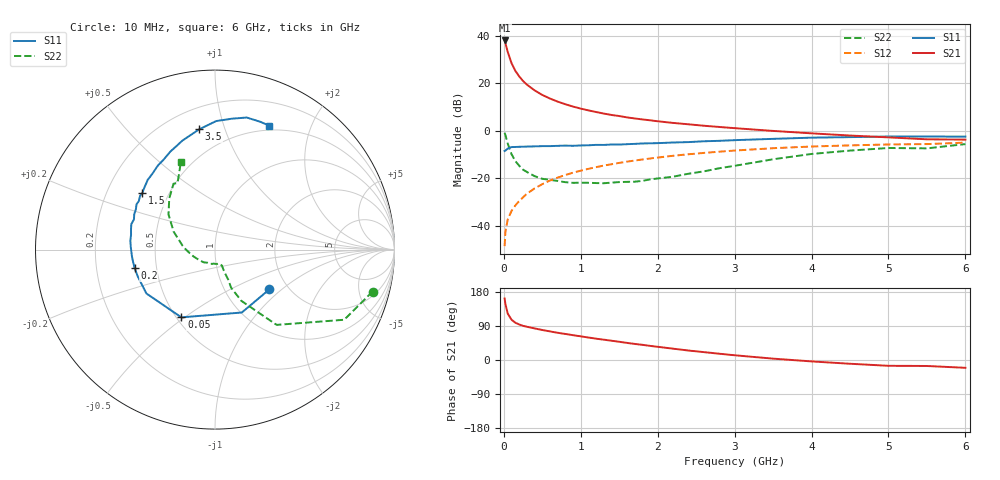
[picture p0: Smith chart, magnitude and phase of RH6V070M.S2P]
! SIEMENS Small Signal Semiconductors
! BFR106
! Si NPN RF Bipolar Junction Transistor in SOT23
! VCE = 6 V  IC = 70 mA
! Common Emitter S-Parameters:  August  1996
# GHz  S  MA  R  50
!  f  S11  S21  S12  S22
! GHz  MAG  ANG  MAG  ANG  MAG  ANG  MAG  ANG
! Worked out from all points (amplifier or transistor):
!   36 points, 10 MHz to 6 GHz, reference 50 ohm
!   highest |S21| = 38.1 dB at 10 MHz (marker M1)
!   |S21| within 3 dB of that: start of sweep to 35.63 MHz
!   unconditionally stable (mu >= 1): 213.4 MHz to 2.336 GHz
!   at 250 MHz: K = 1.03, MAG = 23.4 dB, |S12| = -28.0 dB
!   at 1.4 GHz: K = 1.06, MAG = 8.9 dB, |S12| = -14.1 dB
!   at 6 GHz: K = 0.99, MSG = 0.6 dB, |S12| = -5.0 dB
!   S11 on the Smith chart (normalised r, x): 10 MHz: 1.60, -0.83; 50 MHz: 0.53, -0.49; 200 MHz: 0.37, -0.10; 1.5 GHz: 0.36, +0.30; 3.5 GHz: 0.33, +0.82; 6 GHz: 0.45, +1.43
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0.01  0.3751 -36.3  80.06 162.3  0.0037 78.4  0.9086 -14.9
0.02  0.381 -66.9  71.1 148.2  0.0074 69.0  0.8192 -28.5
0.05  0.4215 -116.4  46.01 122.8  0.0134 61.7  0.542 -50.7
0.1  0.4537 -147.4  26.63 106.3  0.0205 63.0  0.3211 -62.8
0.15  0.4555 -160.7  18.29 98.2  0.0268 66.8  0.2298 -67.1
0.2  0.4595 -167.1  13.95 93.8  0.0332 69.7  0.1832 -66.2
0.25  0.462 -172.2  11.19 90.1  0.0397 70.4  0.1514 -66.9
0.3  0.4644 -175.4  9.369 87.7  0.0472 71.8  0.1354 -67.3
0.4  0.4694 178.3  7.094 83.4  0.0611 73.0  0.1105 -66.9
0.5  0.4744 174.0  5.687 79.2  0.075 73.1  0.0973 -66.4
0.6  0.4749 170.0  4.779 75.5  0.0896 72.3  0.0925 -68.3
0.7  0.4812 166.5  4.118 71.8  0.1032 71.4  0.0876 -71.1
0.9  0.482 159.5  3.235 65.5  0.1309 69.2  0.0799 -76.0
1.1  0.4944 153.1  2.687 59.3  0.1579 66.8  0.0802 -86.3
1.5  0.5125 142.1  2.045 48.1  0.2104 61.2  0.0829 -107.1
1.7  0.5297 136.8  1.82 42.4  0.2359 58.3  0.0845 -119.6
2.2  0.5659 124.3  1.465 29.9  0.2971 50.9  0.1078 -149.0
2.8  0.6142 110.7  1.203 16.6  0.3626 41.8  0.1623 179.7
3.5  0.6758 97.5  0.993 3.6  0.4295 31.5  0.2509 156.6
4.5  0.7352 82.7  0.794 -9.9  0.4922 16.9  0.3825 131.8
5.5  0.7555 70.5  0.661 -15.8  0.5241 7.2  0.4259 119.3
6  0.7539 66.3  0.651 -20.6  0.5629 0.1  0.5237 111.3
